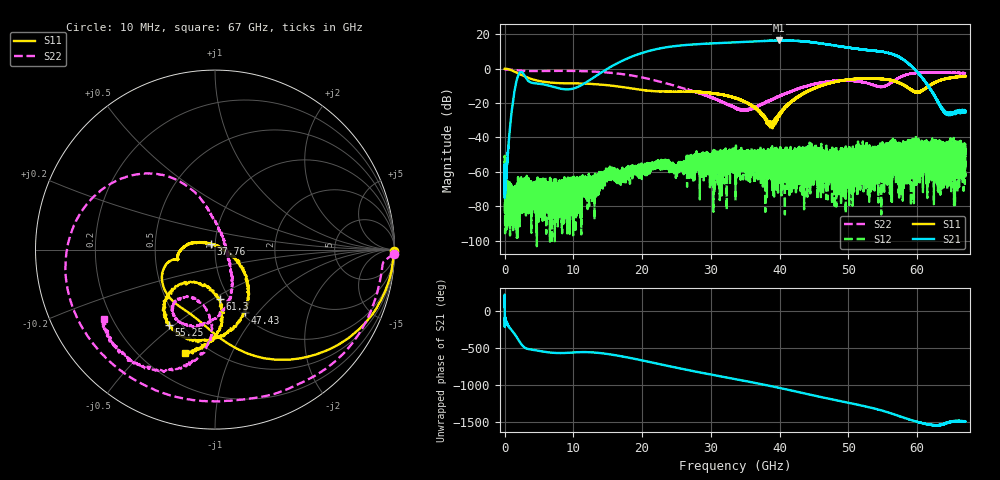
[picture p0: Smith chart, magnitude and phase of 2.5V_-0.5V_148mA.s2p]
! MARKI MICROWAVE INC.
! Date:  10/21/2020
! Model Number:  AMM-7210CH
! Description:  2-port Small Signal S-parameter data for AMM-7210CH
! Frequency Range:  10 MHz to 67 GHz
! Port Configuration:  PORT 1: Input
!  PORT 2: Output
! Bias Condition: Vd = +2.5V, Vg = -0.5V
! AMM-7210CH s2p files are only valid for small signal conditions (below -10 dBm input power)
# Hz S  dB  R 50
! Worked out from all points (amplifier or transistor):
!   20001 points, 10 MHz to 67 GHz, reference 50 ohm
!   highest |S21| = 16.3 dB at 39.96 GHz (marker M1)
!   |S21| within 3 dB of that: 25.43 GHz to 48.01 GHz (22.59 GHz wide, 61.5 % of centre)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
!   unconditionally stable (mu >= 1): start of sweep to 10.00715 MHz; 16.68 MHz to end of sweep
!   at 11.17 GHz: K = 708.93, MAG = -3.5 dB, |S12| = -65.6 dB
!   at 33.51 GHz: K = 48.39, MAG = 15.4 dB, |S12| = -55.2 dB
!   at 67 GHz: K = 2001.65, MAG = -20.1 dB, |S12| = -57.2 dB
!   S11 on the Smith chart (normalised r, x): 10 MHz: open; 37.76 GHz: 0.96, +0.06; 47.43 GHz: 1.04, -0.86; 55.25 GHz: 0.43, -0.48; 61.3 GHz: 0.90, -0.54; 67 GHz: 0.39, -0.66
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1e7  -0.03 -0.5  -63.15 45.8  -61.85 -38.1  -0.04 -1.4
2.203922e9  -3.19 -62.1  -2.31 -60.3  -71.64 34.4  -1.14 -61.1
1.117723e10  -8.68 -133.3  -9.62 161.4  -71.53 -158.0  -1.46 -169.4
1.696182e10  -10.66 -161.7  4.23 105.6  -62.64 127.9  -3.12 149.4
1.987254e10  -12.34 -166.4  8.91 52.3  -60.32 133.8  -5.03 130.8
2.234112e10  -13.26 -165.0  11.52 3.6  -55.04 102.4  -7.34 117.6
2.473601e10  -13.48 -165.3  13.05 -43.4  -58.81 69.3  -9.95 107.5
2.781755e10  -13.53 -170.0  14.12 -101.2  -54.42 80.8  -13.66 97.7
3.095938e10  -14.73 178.0  14.78 -157.1  -54.83 56.2  -18.22 82.5
3.3505e10  -16.93 165.9  15.27 158.4  -55.21 26.3  -22.74 49.6
3.588314e10  -21.31 153.2  15.73 116.6  -51.47 2.8  -23.14 -11.1
3.776221e10  -28.40 124.5  16.03 81.8  -60.85 -30.1  -20.02 -37.4
3.995614e10  -26.36 4.5  16.35 40.0  -49.45 -88.9  -15.93 -55.5
4.223715e10  -17.51 -26.0  16.17 -6.1  -52.63 -65.2  -12.37 -67.4
4.467223e10  -12.15 -43.3  15.38 -56.3  -54.82 122.0  -9.38 -82.8
4.743222e10  -8.23 -64.5  13.76 -111.0  -62.86 -26.8  -7.40 -100.8
5.106978e10  -6.02 -92.5  11.56 178.5  -50.51 -107.3  -7.25 -121.4
5.52533e10  -6.13 -121.6  9.58 84.5  -53.53 -169.2  -10.26 -105.9
5.583612e10  -6.49 -124.7  9.07 68.0  -62.63 -146.6  -9.10 -97.8
5.86162e10  -11.07 -136.3  3.29 -17.9  -49.29 -79.4  -3.37 -105.6
6.129915e10  -11.16 -84.4  -8.46 -86.6  -44.91 145.6  -2.12 -124.9
6.7e10  -4.60 -107.2  -25.38 -53.0  -57.17 -60.8  -2.65 -148.5
